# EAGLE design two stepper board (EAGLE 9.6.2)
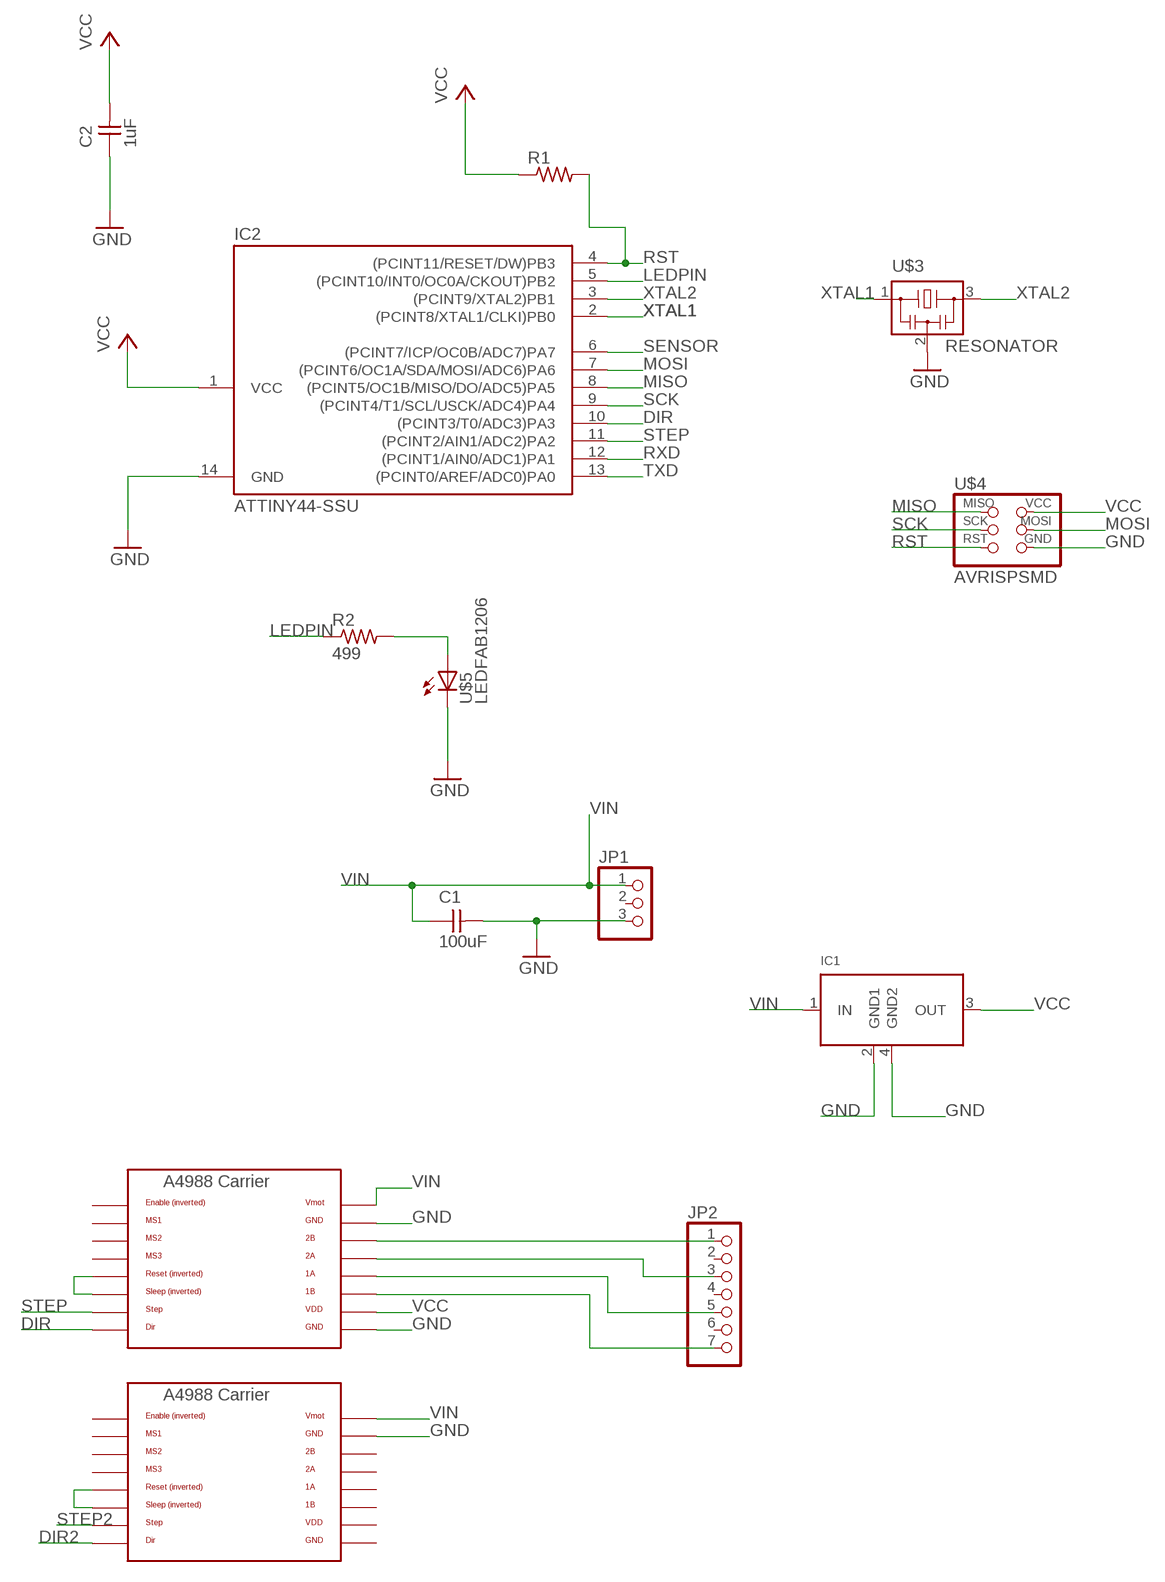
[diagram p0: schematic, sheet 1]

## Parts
C1  100uF  CAP-UNPOLARIZEDFAB  [C1206FAB]
C2  1uF  CAP-UNPOLARIZEDFAB  [C1206FAB]
IC1  VREG_MULTI  [SOT223]
IC2  ATTINY44-SSU  [SOIC14]
JP1  PINHD-1X3  [1X03]
JP2  PINHD-1X7  [1X07]
R1  RES-US1206FAB  [R1206FAB]
R2  499  RES-US1206FAB  [R1206FAB]
U$1  A4983CARRIER  [A4988BREAKOUT]
U$3  RESONATOR  [EFOBM]
U$4  AVRISPSMD  [2X03SMD]
U$5  LEDFAB1206  [LED1206FAB]
U$6  A4988BREAKOUT  [A4988BREAKOUT]

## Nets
DIR: IC2.10((PCINT3/T0/ADC3)PA3) U$1.DIR
DIR2: U$6.DIR
GND: C1.2 C2.1 IC1.2(GND1) IC1.4(GND2) IC2.14(GND) JP1.3 U$1.GND(GNDMOT) U$1.GND@0(GND) U$3.2 U$4.6(GND) U$5.2(C) U$6.GND@0(GNDMOT)
LEDPIN: IC2.5((PCINT10/INT0/OC0A/CKOUT)PB2) R2.1
MISO: IC2.8((PCINT5/OC1B/MISO/DO/ADC5)PA5) U$4.1(MISO)
MOSI: IC2.7((PCINT6/OC1A/SDA/MOSI/ADC6)PA6) U$4.4(MOSI)
N$1: JP2.1 U$1.2B
N$2: JP2.3 U$1.2A
N$3: JP2.5 U$1.1A
N$4: JP2.7 U$1.1B
N$5: U$1.RST U$1.SLP(SLEEP)
N$6: R2.2 U$5.1(A)
N$8: U$6.RST U$6.SLP(SLEEP)
RST: IC2.4((PCINT11/RESET/DW)PB3) R1.2 U$4.5(RST)
RXD: IC2.12((PCINT1/AIN0/ADC1)PA1)
SCK: IC2.9((PCINT4/T1/SCL/USCK/ADC4)PA4) U$4.3(SCK)
SENSOR: IC2.6((PCINT7/ICP/OC0B/ADC7)PA7)
STEP: IC2.11((PCINT2/AIN1/ADC2)PA2) U$1.STEP
STEP2: U$6.STEP
TXD: IC2.13((PCINT0/AREF/ADC0)PA0)
VCC: C2.2 IC1.3(OUT) IC2.1(VCC) R1.1 U$1.VDD U$4.2(VCC)
VIN: C1.1 IC1.1(IN) JP1.1 U$1.VMOT U$6.VMOT
XTAL1: IC2.2((PCINT8/XTAL1/CLKI)PB0) U$3.1
XTAL2: IC2.3((PCINT9/XTAL2)PB1) U$3.3
Unconnected: JP1.2 JP2.2 JP2.4 JP2.6 U$1.EN U$1.MS1 U$1.MS2 U$1.MS3 U$6.1A U$6.1B U$6.2A U$6.2B U$6.EN U$6.MS1 U$6.MS2 U$6.MS3

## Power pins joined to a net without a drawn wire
GND: U$6.GND
VDD: U$6.VDD

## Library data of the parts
C1 C2 = fab:CAP-UNPOLARIZED
IC1 = m-pad-2.1:VREG_MULTI: standard package voltage regulator (LM2940, LM2937, LM340, UA78M05, etc)
IC2 = fab:ATTINY44
JP1 = pinhead:PINHD-1X3: PIN HEADER
JP2 = pinhead:PINHD-1X7: PIN HEADER
R1 R2 = fab:RES-US: Resistor (US Symbol)
U$1 = RepRapjr:A4983CARRIER
U$3 = fab:RESONATOR
U$4 = fab:AVRISP
U$5 = fab:LED: LED
U$6 = RepRapjr:A4988BREAKOUT

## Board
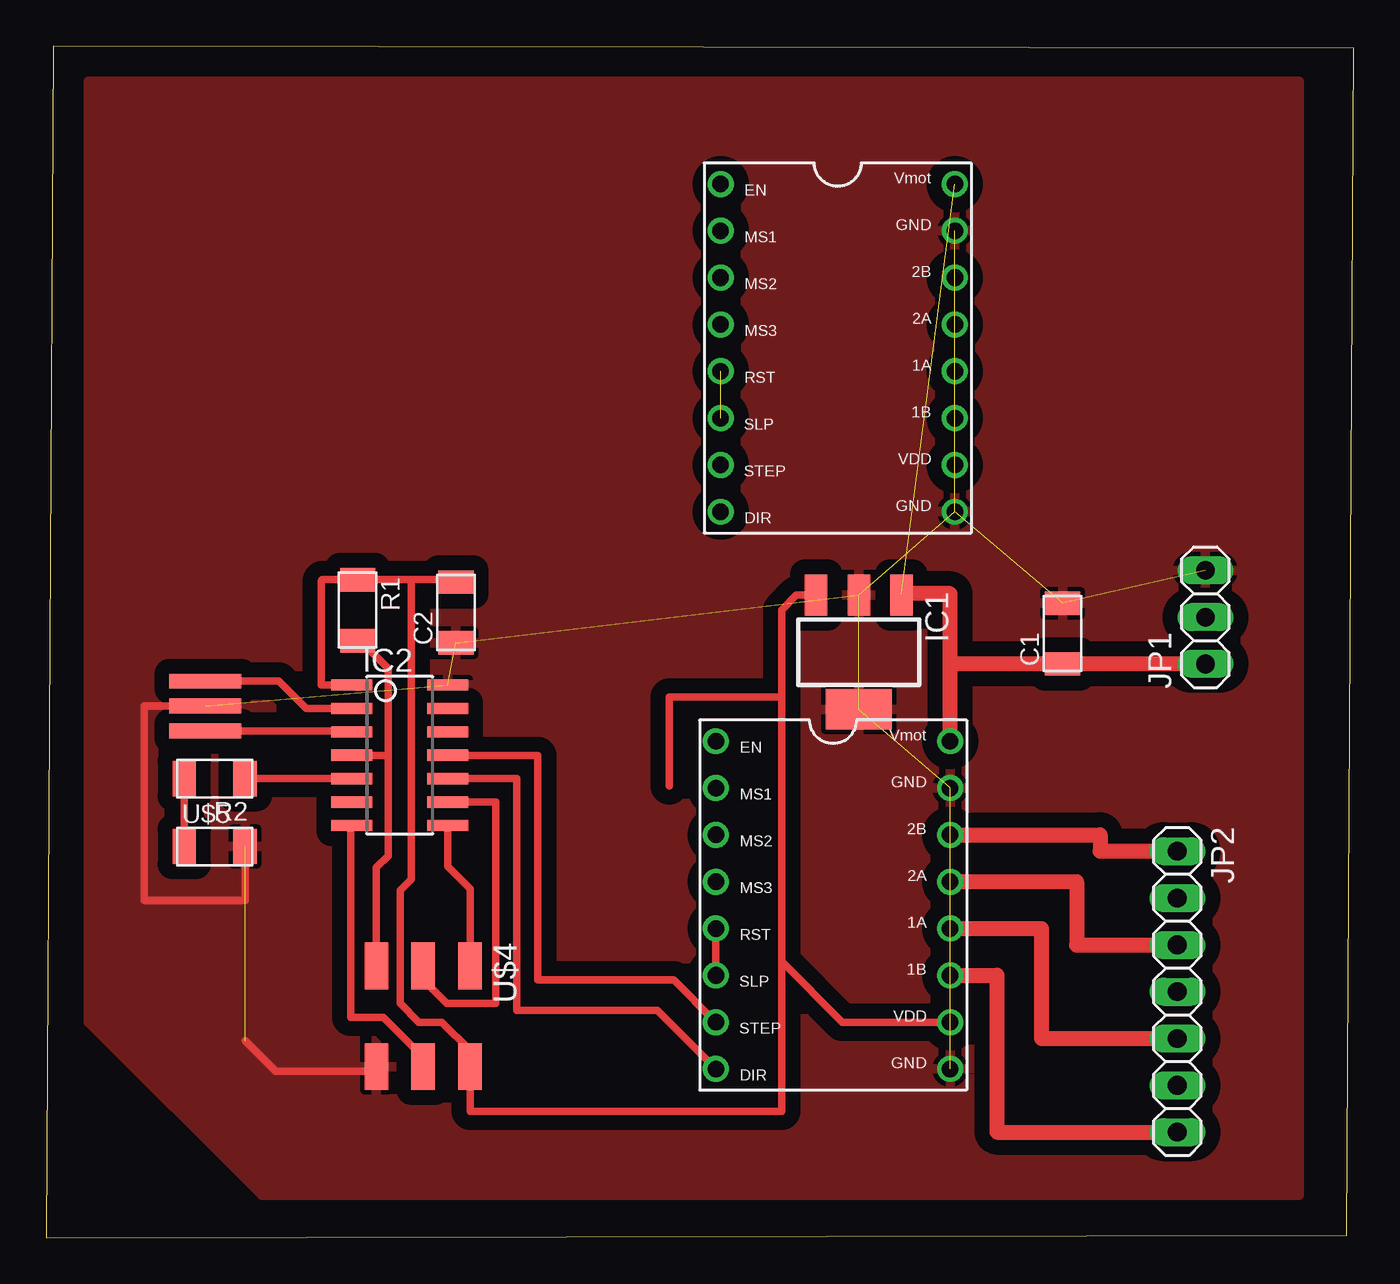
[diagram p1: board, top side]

Size 70.92 x 64.63 mm. Coordinates in mm from the lower left corner, seen from the top.
Outline: 0,0 70.54,0.13 70.92,64.51 0.38,64.63 0,0
Copper layers (1*16): Top 0.035mm / dielectric 1.5mm / Bottom 0.035mm
Design rules "default *": minimum track width 6mil, minimum drill 0.35mm, track to track 16mil, track to pad 16mil, pad to pad 6mil, via to via 6mil, smd to smd 6mil, copper to edge 40mil, drill to drill 6mil, minimum pad ring 10mil, minimum via ring 8mil, stop-mask expansion 4mil, vias tented up to drill 0mil, thermal gap 10mil

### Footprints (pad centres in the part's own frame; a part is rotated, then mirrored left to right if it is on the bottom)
C1206FAB = smd 1.27 x 1.905: 1 -1.651,0; 2 1.651,0
SOT223 = smd 1.219 x 2.235: 1 -2.311,-3.099; 2 0,-3.099; 3 2.311,-3.099 | smd 3.6 x 2.2: 4 0,3.099
SOIC14 = smd 0.61 x 2.21: 1 -3.81,-2.603; 2 -2.54,-2.603; 3 -1.27,-2.603; 4 0,-2.603; 5 1.27,-2.603; 6 2.54,-2.603; 7 3.81,-2.603; 8 3.81,2.603; 9 2.54,2.603; 10 1.27,2.603; 11 0,2.603; 12 -1.27,2.603; 13 -2.54,2.603; 14 -3.81,2.603
1X03 = drill 1.016 long: 1 -2.54,0; 2 0,0; 3 2.54,0
1X07 = drill 1.016 long: 1 -7.62,0; 2 -5.08,0; 3 -2.54,0; 4 0,0; 5 2.54,0; 6 5.08,0; 7 7.62,0
R1206FAB = smd 1.27 x 1.905: 1 -1.651,0; 2 1.651,0
A4988BREAKOUT = drill 0.9: 1A 8.89,1.27; 1B 11.43,1.27; 2A 6.35,1.27; 2B 3.81,1.27; DIR 16.51,-11.43; EN -1.27,-11.43; GND 16.51,1.27; GND@0 1.27,1.27; MS1 1.27,-11.43; MS2 3.81,-11.43; MS3 6.35,-11.43; RST 8.89,-11.43; SLP 11.43,-11.43; STEP 13.97,-11.43; VDD 13.97,1.27; VMOT -1.27,1.27
EFOBM = smd 0.8 x 3.9: 1 -1.35,0; 2 0,0; 3 1.35,0
2X03SMD = smd 2.54 x 1.27: 1 -2.54,2.54; 2 2.92,2.54; 3 -2.54,0; 4 2.92,0; 5 -2.54,-2.54; 6 2.92,-2.54
LED1206FAB = smd 1.27 x 1.905: 1 -1.651,0; 2 1.651,0

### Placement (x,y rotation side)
C1  55.12,32.77 90 top
C2  22.23,33.91 90 top
IC1  44.07,31.75 180 top
IC2  19.18,26.16 270 top
JP1  62.86,33.66 90 top
JP2  61.34,13.33 270 top
R1  16.89,34.04 270 top
R2  9.14,24.89 180 top
U$1  47.75,25.65 270 top
U$3  8.64,28.83 270 top
U$4  20.45,12.19 270 top
U$5  9.14,21.21 0 top
U$6  48.01,55.88 270 top

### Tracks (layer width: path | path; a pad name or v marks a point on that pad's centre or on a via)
DIR
  Top 0.406: IC2.10 25.53,24.89 25.53,12.32 33.15,12.32 U$1.DIR
GND  (11 unrouted)
  Top 0.406: U$4.6 17.65,9.02 12.45,9.02 10.8,10.67 | U$5.2 10.8,18.29 5.33,18.29 5.33,28.83 U$3.2
  pour Top (isolate 0.813): 67.95,2.29 11.68,2.29 2.29,11.68 2.29,62.74 67.95,62.74
LEDPIN
  Top 0.406: IC2.5 R2.1
MISO
  Top 0.406: IC2.8 21.78,20.13 22.99,18.92 U$4.1
MOSI
  Top 0.406: IC2.7 16.51,22.29 16.51,11.94 18.29,11.94 20.45,9.78 U$4.4
N$1
  Top 0.813: 60.71,20.95 JP2.1 57.15,20.95 57.15,21.84 U$1.2B
N$2
  Top 0.813: 60.96,15.87 JP2.3 55.88,15.87 55.88,19.3 U$1.2A
N$3
  Top 0.813: U$1.1A 53.97,16.76 53.97,10.79 JP2.5
N$4
  Top 0.813: U$1.1B 51.56,14.22 51.56,5.71 JP2.7
N$5
  Top 0.406: U$1.RST U$1.SLP
N$6
  Top 0.406: R2.2 U$5.1
N$8  (1 unrouted)
RST
  Top 0.406: IC2.4 18.54,26.16 | 18.54,26.16 18.54,20.7 17.91,20.07 U$4.5 | 18.54,26.16 18.54,30.86 17.02,32.38 R1.2
SCK
  Top 0.406: IC2.9 24.38,23.62 24.38,12.7 21.72,12.7 20.45,13.97 U$4.3
STEP
  Top 0.406: IC2.11 26.67,26.16 26.67,13.97 34.04,13.97 U$1.STEP
VCC
  Top 0.406: IC2.1 14.92,29.97 14.92,35.62 14.99,35.69 R1.1 19.81,35.69 | 39.88,14.99 39.88,6.86 22.99,6.86 U$4.2 22.99,10.16 21.46,11.68 20.22,11.68 19.2,12.7 19.2,18.82 19.81,19.43 19.81,35.69 | 39.88,14.99 39.88,29.34 | 33.78,24.51 33.78,29.34 39.88,29.34 | U$1.VDD 43.18,11.68 39.88,14.99 | 19.81,35.69 22.1,35.69 C2.2 | 39.88,29.34 39.88,34.04 40.69,34.85 IC1.3
VIN  (1 unrouted)
  Top 0.813: JP1.1 C1.1 49.02,31.11 | U$1.VMOT 49.02,31.11 | 49.02,31.11 49.02,34.92 46.38,34.92 IC1.1
XTAL1
  Top 0.406: IC2.2 14.1,28.7 12.62,30.18 U$3.1
XTAL2
  Top 0.406: IC2.3 16.53,27.48 U$3.3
